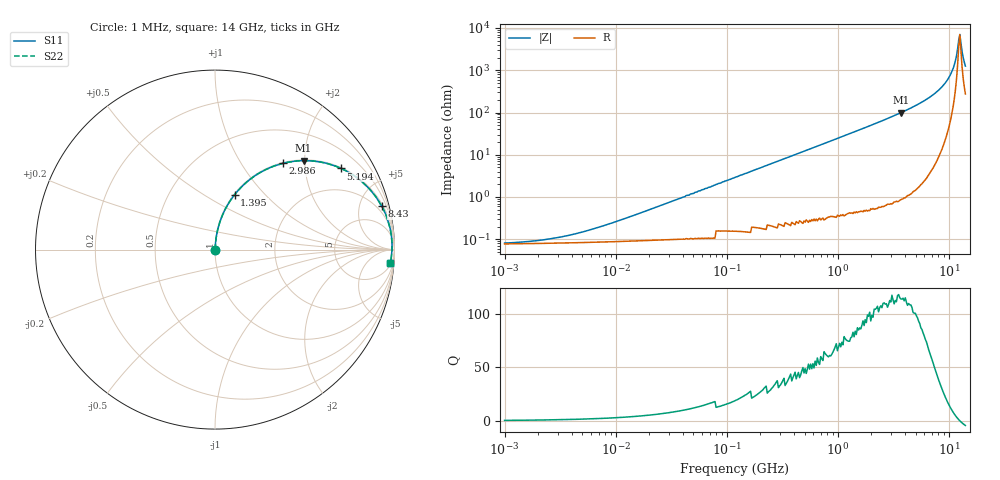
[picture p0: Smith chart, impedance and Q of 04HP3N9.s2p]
# MHz S MA R 50
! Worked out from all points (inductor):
!   415 points, 1 MHz to 14 GHz, reference 50 ohm
!   read as one part in series: L = 3.9 nH near 11 MHz
!   highest Q = 115 at 3.675 GHz (marker M1), where L = 4.27 nH
!   self-resonance near 12.19 GHz
!   S11 on the Smith chart (normalised r, x): 1 MHz: 1.00, +0.00; 1.395 GHz: 1.01, +0.69; 2.986 GHz: 1.01, +1.55; 5.194 GHz: 1.03, +3.08; 8.43 GHz: 1.24, +7.63; 14 GHz: 7, -25
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1  0.0005991 24.1  0.999 -0.0  0.999 -0.0  0.0005991 24.1
2.294  0.0008194 43.2  0.999 -0.0  0.999 -0.0  0.0008194 43.2
5.024  0.001399 61.5  0.999 -0.1  0.999 -0.1  0.001399 61.5
24.664  0.006109 80.9  0.999 -0.3  0.999 -0.3  0.006109 80.9
118.322  0.029 85.4  0.998 -1.7  0.998 -1.7  0.029 85.4
580.879  0.141 80.8  0.987 -8.1  0.987 -8.1  0.141 80.8
1395.237  0.326 70.3  0.941 -19.0  0.941 -19.0  0.326 70.3
2851.719  0.591 53.3  0.801 -36.2  0.801 -36.2  0.591 53.3
2986.32  0.611 51.9  0.786 -37.6  0.786 -37.6  0.611 51.9
3675.103  0.699 45.1  0.709 -44.4  0.709 -44.4  0.699 45.1
5193.876  0.835 32.8  0.542 -56.6  0.542 -56.6  0.835 32.8
6849.662  0.918 22.4  0.381 -66.7  0.381 -66.7  0.918 22.4
8429.511  0.96 14.6  0.252 -73.7  0.252 -73.7  0.96 14.6
9680.353  0.977 9.4  0.163 -77.4  0.163 -77.4  0.977 9.4
10615.74  0.984 5.9  0.103 -78.1  0.103 -78.1  0.984 5.9
11116.81  0.986 4.2  0.074 -76.8  0.074 -76.8  0.986 4.2
11913.09  0.987 1.6  0.031 -63.8  0.031 -63.8  0.987 1.6
12191  0.986 0.8  0.019 -44.0  0.019 -44.0  0.986 0.8
12475.39  0.986 -0.1  0.014 6.3  0.014 6.3  0.986 -0.1
12766.41  0.985 -0.9  0.022 47.7  0.022 47.7  0.985 -0.9
13680.85  0.982 -3.5  0.063 71.5  0.063 71.5  0.982 -3.5
14000  0.98 -4.3  0.078 73.0  0.078 73.0  0.98 -4.3
